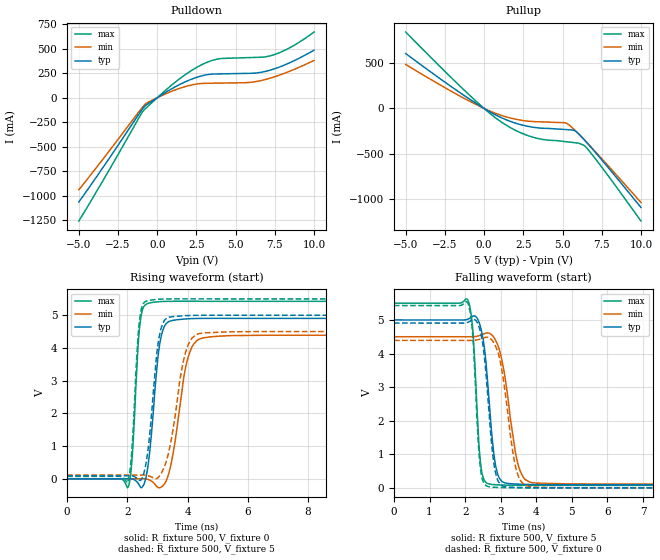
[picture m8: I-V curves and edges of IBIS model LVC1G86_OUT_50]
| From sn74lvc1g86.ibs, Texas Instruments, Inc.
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[Model]   LVC1G86_OUT_50
Model_type  Output
Vref =   0
Rref =   500
Cref =   50p
Vmeas =   2.5
| variable   typ   min   max
C_comp   8.87pF   5.48pF   12.17pF
| C_pullup   9.50pF   5.48pF   12.17pF
| C_pulldown   8.23pF   6.09pF   11.09pF
[Temperature Range]   40   100   -40
| Ambient temperature   25   85   -40
[Voltage range]   5   4.5   5.5
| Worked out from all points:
|   slope of the pulldown table from 0 to 0.75 V, typ, clamps not added: 9.96 ohm
|   slope of the pullup table from 0 to 0.75 V, typ, clamps not added: 10.3 ohm
|   rising waveform, R_fixture 500, V_fixture 0: 20-80 % time 285ps typ, 422ps min, 188ps max; typ from 0 V to 4.9 V
|   falling waveform, R_fixture 500, V_fixture 5: 20-80 % time 242ps typ, 358ps min, 163ps max; typ from 5 V to 0.093 V
|   rising waveform, R_fixture 500, V_fixture 5: 20-80 % time 293ps typ, 453ps min, 190ps max; typ from 0.093 V to 5 V
|   falling waveform, R_fixture 500, V_fixture 0: 20-80 % time 239ps typ, 338ps min, 159ps max; typ from 4.91 V to 0 V
[Pulldown]
| LVC1G86_OUT_50
|   Voltage   I(typ)   I(min)   I(max)
-5V       -1.064A    -939.9mA   -1.259A
-3.38V    -693.4mA   -609.7mA   -824.1mA
-925mV    -111.5mA   -93.72mA   -140.8mA
-625mV    -66.36mA   -49.46mA   -92.33mA
1.08V     105.5mA    75.95mA    149.9mA
2.29V     195.8mA    133.5mA    288.3mA
3.34V     238.7mA    148.2mA    372.1mA
4.085V    243.6mA    149.9mA    400.5mA
5.84V     249.3mA    155.7mA    409.9mA
7.285V    285.8mA    204mA      431.5mA
8.51V     361.9mA    274.7mA    515.7mA
10V       485.6mA    380.4mA    671mA
[Pullup]
| LVC1G86_OUT_50
|   Voltage   I(typ)   I(min)   I(max)
-5V       604.5mA    484.9mA    841.8mA
-1.075V   119.7mA    93.33mA    170.1mA
205mV     -21.37mA   -16.3mA    -30.84mA
1.085V    -100.6mA   -75.34mA   -147.2mA
2.055V    -164.7mA   -120mA     -245.4mA
3.025V    -204.3mA   -143.2mA   -312mA
3.86V     -218.8mA   -148.7mA   -344.2mA
5.29V     -233.1mA   -166mA     -367.5mA
5.825V    -248.5mA   -246.3mA   -378.1mA
6.49V     -363.8mA   -364.3mA   -425.1mA
7.725V    -612.1mA   -595.8mA   -697.9mA
10V       -1.09A     -1.035A    -1.24A
[Ramp]
| LVC1G86_OUT_50
| variable   typ   min   max
dV/dt_r   3.10/3.12E-10   2.80/4.68E-10   3.42/2.05E-10
dV/dt_f   3.01/2.52E-10   2.70/3.81E-10   3.33/1.73E-10
R_load = 500
[Rising Waveform]
| LVC1G86_OUT_50
R_fixture =   500
C_fixture =   0
L_fixture =   0
V_fixture =   0
V_fixture_min = 0
V_fixture_max = 0
|   Time   V(typ)   V(min)   V(max)
0s        187.4pV    4.423nV    603.7pV
2.03ns    1.958mV    -80.02uV   -250.8mV
2.16ns    -4.012mV   4.932uV    649.3mV
2.445ns   -269.3mV   3.076mV    4.908V
2.685ns   389.3mV    -18.58mV   5.364V
2.915ns   2.699V     -165mV     5.403V
3.275ns   4.729V     -89.19mV   5.424V
4.02ns    4.892V     3.72V      5.428V
4.73ns    4.905V     4.338V     5.427V
50ns      4.904V     4.387V     5.427V
[Falling Waveform]
| LVC1G86_OUT_50
R_fixture =   500
C_fixture =   0
L_fixture =   0
V_fixture =   5
V_fixture_min = 4.5
V_fixture_max = 5.5
|   Time   V(typ)   V(min)   V(max)
0s        5V         4.5V       5.5V
2.075ns   5.021V     4.497V     5.593V
2.215ns   5.113V     4.498V     4.706V
2.45ns    4.718V     4.552V     594.9mV
2.575ns   3.852V     4.604V     170.8mV
2.76ns    1.478V     4.544V     98.93mV
2.955ns   300.5mV    4.139V     87.31mV
3.5ns     110.2mV    648.5mV    75mV
3.98ns    96.84mV    142.2mV    73.25mV
50ns      92.93mV    112.7mV    73.54mV
[Rising Waveform]
| LVC1G86_OUT_50
R_fixture =   500
C_fixture =   0
L_fixture =   0
V_fixture =   5
V_fixture_min = 4.5
V_fixture_max = 5.5
|   Time   V(typ)   V(min)   V(max)
0s        92.92mV    112.6mV    73.53mV
2.01ns    94.42mV    112.6mV    -104.8mV
2.145ns   91.32mV    112.6mV    810.6mV
2.42ns    -47.74mV   115.1mV    4.944V
2.66ns    700.9mV    102.4mV    5.441V
2.89ns    2.946V     24.12mV    5.477V
3.245ns   4.859V     402.8mV    5.497V
3.94ns    4.987V     3.886V     5.501V
4.545ns   5.001V     4.461V     5.5V
50ns      5V         4.5V       5.5V
[Falling Waveform]
| LVC1G86_OUT_50
R_fixture =   500
C_fixture =   0
L_fixture =   0
V_fixture =   0
V_fixture_min = 0
V_fixture_max = 0
|   Time   V(typ)   V(min)   V(max)
0s        4.907V     4.391V     5.429V
2.07ns    4.926V     4.388V     5.514V
2.21ns    5.007V     4.39V      4.601V
2.435ns   4.622V     4.433V     544.7mV
2.55ns    3.805V     4.475V     105.3mV
2.75ns    1.24V      4.404V     20.69mV
2.935ns   184.1mV    3.984V     11.24mV
3.445ns   12.78mV    511.1mV    1.621mV
3.935ns   3.333mV    22.7mV     -129.9uV
50ns      8.33uV     13.18uV    5.644uV
